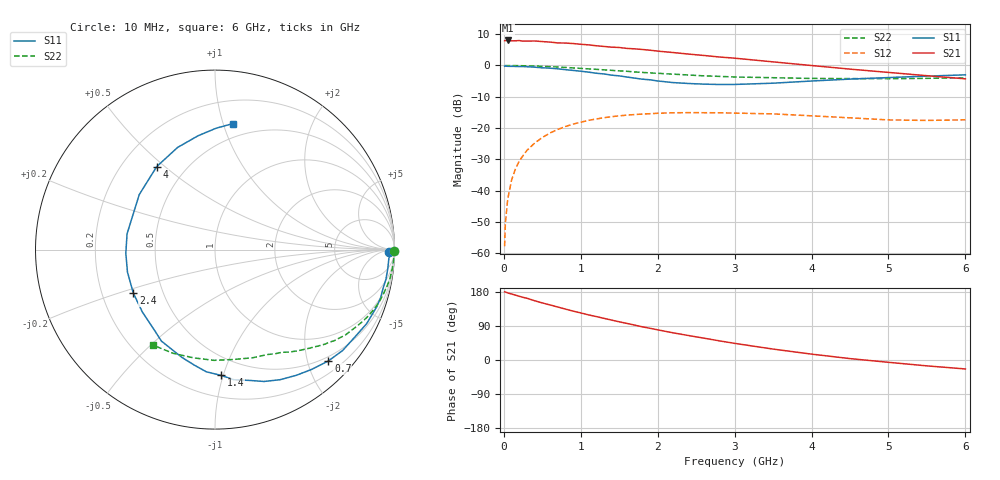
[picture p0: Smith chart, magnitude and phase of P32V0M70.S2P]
! SIEMENS Small Signal Semiconductors
! BFP181
! Si NPN RF Bipolar Junction Transistor in SOT143
! VCE = 2 V  IC = 0.7 mA
! Common Emitter S-Parameters:  March  1996
# GHz  S  MA  R  50
!  f  S11  S21  S12  S22
! GHz  MAG  ANG  MAG  ANG  MAG  ANG  MAG  ANG
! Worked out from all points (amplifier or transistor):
!   36 points, 10 MHz to 6 GHz, reference 50 ohm
!   highest |S21| = 8.0 dB at 50 MHz (marker M1)
!   |S21| within 3 dB of that: start of sweep to 1.85 GHz
!   unconditionally stable (mu >= 1): 3.485 GHz to end of sweep
!   at 250 MHz: K = 0.08, MSG = 18.3 dB, |S12| = -28.8 dB
!   at 1.4 GHz: K = 0.46, MSG = 11.1 dB, |S12| = -16.4 dB
!   at 6 GHz: K = 1.39, MAG = 2.8 dB, |S12| = -17.4 dB
!   S11 on the Smith chart (normalised r, x): 10 MHz: 59, -26; 700 MHz: 0.42, -2.38; 1.4 GHz: 0.36, -0.98; 2.4 GHz: 0.34, -0.22; 4 GHz: 0.35, +0.47; 6 GHz: 0.38, +1.08
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0.01  0.972 -0.7  2.488 179.8  0.0013 92.0  0.9988 -0.3
0.02  0.9782 -1.3  2.491 179.5  0.003 82.2  0.993 -0.5
0.05  0.97 -2.9  2.511 177.1  0.0073 89.5  0.9977 -1.6
0.1  0.9685 -6.4  2.479 174.2  0.0147 84.6  0.9971 -3.1
0.15  0.9667 -9.9  2.482 171.2  0.0222 82.8  0.9945 -4.6
0.2  0.9608 -13.1  2.501 168.2  0.0297 81.2  0.9936 -6.2
0.25  0.961 -16.2  2.451 165.3  0.0364 79.3  0.9898 -7.7
0.4  0.9405 -26.0  2.463 156.4  0.0575 72.5  0.9799 -12.2
0.7  0.8853 -44.5  2.294 139.9  0.0952 59.7  0.945 -20.7
0.9  0.8341 -57.1  2.242 129.1  0.1157 51.5  0.9148 -25.9
1.1  0.7838 -69.6  2.136 119.1  0.1328 44.4  0.8826 -30.7
1.4  0.7014 -87.3  1.962 105.4  0.1522 34.6  0.8368 -37.3
1.5  0.6824 -94.1  1.939 100.8  0.1568 31.9  0.8197 -39.0
1.8  0.6046 -113.8  1.802 87.5  0.1675 24.1  0.7755 -44.3
2.2  0.5334 -139.4  1.61 71.7  0.1756 14.7  0.7272 -50.9
2.4  0.5158 -151.9  1.522 64.6  0.1766 10.4  0.7047 -54.1
3  0.4978 169.8  1.309 43.9  0.1737 0.3  0.6549 -63.1
3.5  0.5216 144.0  1.142 28.8  0.1686 -5.6  0.638 -70.8
4  0.565 125.1  0.999 15.5  0.157 -10.1  0.6212 -80.1
4.5  0.6062 110.1  0.875 3.7  0.1459 -12.5  0.6171 -90.5
5.5  0.6762 89.5  0.687 -15.5  0.1326 -8.5  0.6234 -112.0
6  0.7092 81.9  0.612 -23.6  0.1356 -5.5  0.6345 -123.1
